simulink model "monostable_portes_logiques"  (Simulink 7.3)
settings: Solver=ode15s  StartTime=0.0  StopTime=1  RelTol=1e-3
StopFcn:
  | close all, clc
  | load signaux.mat
  | plot(x(1,:),x(2,:))
  | grid
  | title('Oscillateur à portes NAND, T=2RC ln3')
  | 
  | xlabel('temps')
  | axis([0 1 -0.1 1.1])
undefined symbols (not defined in the file or in its folder): sigbuilder_block
libraries: fl_lib x6, elec_lib x5, nesl_utility x4

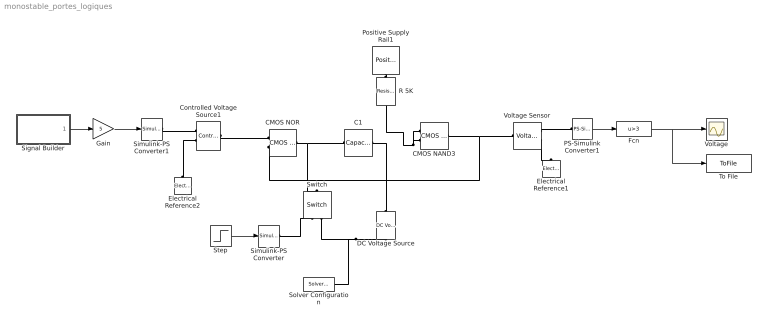
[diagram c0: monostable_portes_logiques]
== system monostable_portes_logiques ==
  C1 : fl_lib/Electrical/Electrical Elements/Capacitor  DialogController=NetworkEngine.DynNeDlgSource  SystemSampleTime=-1  c=100e-9 F  v0=0 V  r=1e-6 Ohm  g=0 1/Ohm  i_Log=off  v_Log=off  vc_Log=off  LocalVarNames=|current|voltage|power  LocalVarDescs=|Capacitor current (A)|Voltage across capacitor (V)|Power (W)  LocalVarLogging=[0 0 0]
  CMOS NAND3 : elec_lib/Integrated Circuits/Logic/CMOS NAND  DialogController=NetworkEngine.DynNeDlgSource  SystemSampleTime=-1  V_IL=2 V  V_IH=3 V  V_OL=0 V  V_OH=5 V  C_IN=5 pF  R_OUT=450 Ohm  Delay=1.2e-07 s  LocalVarLogging=[]
  CMOS NOR : elec_lib/Integrated Circuits/Logic/CMOS NOR  DialogController=NetworkEngine.DynNeDlgSource  SystemSampleTime=-1  V_IL=2 V  V_IH=3 V  V_OL=0 V  V_OH=5 V  C_IN=5 pF  R_OUT=450 Ohm  Delay=1.2e-07 s  LocalVarLogging=[]
  Controlled Voltage Source1 : fl_lib/Electrical/Electrical Sources/Controlled Voltage Source  DialogController=NetworkEngine.DynNeDlgSource  SystemSampleTime=-1  i_Log=off  v_Log=off  LocalVarNames=|current|voltage|power  LocalVarDescs=|Current (A)|Voltage (V)|Power (W)  LocalVarLogging=[0 0 0]
  DC Voltage Source : elec_lib/Sources/SPICE-Compatible Sources/DC Voltage Source  DialogController=NetworkEngine.DynNeDlgSource  SystemSampleTime=-1  DC=1 V  current_Log=off  voltage_Log=off  power_Log=off  LocalVarNames=|current|voltage|power  LocalVarDescs=|Current (A)|Voltage (V)|Power (W)  LocalVarLogging=[0 0 0]
  Electrical Reference1 : fl_lib/Electrical/Electrical Elements/Electrical Reference  DialogController=NetworkEngine.DynNeDlgSource  SystemSampleTime=-1  i_Log=off  LocalVarNames=|i  LocalVarDescs=|i  LocalVarLogging=[]
  Electrical Reference2 : fl_lib/Electrical/Electrical Elements/Electrical Reference  DialogController=NetworkEngine.DynNeDlgSource  SystemSampleTime=-1  i_Log=off  LocalVarNames=|i  LocalVarDescs=|i  LocalVarLogging=[]
  Fcn : Fcn  Expr=u>3
  Gain : Gain  Gain=5  ParameterDataType=fixdt(1, 16)  ParameterScaling=2^0  OutDataType=fixdt(1, 16)  OutScaling=2^0
  PS-Simulink Converter1 : nesl_utility/PS-Simulink Converter  DialogController=NetworkEngine.DynNeUtilDlgSource  SystemSampleTime=-1  PhysicalDomain=network_engine_domain  LeftPortType=input  RightPortType=output  SubClassName=ps_output  Unit=1  AffineConversion=off
  Positive Supply Rail1 : elec_lib/Sources/Positive Supply Rail  DialogController=NetworkEngine.DynNeDlgSource  SystemSampleTime=-1  v0=5 V  current_Log=off  voltage_Log=off  power_Log=off  LocalVarNames=|current|voltage|power  LocalVarDescs=|Current (A)|Voltage (V)|Power (W)  LocalVarLogging=[0 0 0]
  R 5K : elec_lib/Passive Devices/Resistor  DialogController=NetworkEngine.DynNeDlgSource  SystemSampleTime=-1  SCALE=1  R_param=1  R=5 kOhm  RSH=0 Ohm  LENGTH=1e-06 m  WIDTH=1e-06 m  NARROW=0 m  T_param=1  TC1=0 1/K  TC2=0 1/K^2  TOFFSET=0 K  TFIXED=300.15 K  TMEAS=300.15 K  LocalVarLogging=[]
  Signal Builder : Subsystem  Tag=STV Subsys  LoadFcn=sigbuilder_block('load',[198 37.5 550.5 399.75 ]);  StartFcn=sigbuilder_block('start');  StopFcn=sigbuilder_block('stop');  ClipboardFcn=sigbuilder_block('clipboard');
  Simulink-PS Converter : nesl_utility/Simulink-PS Converter  DialogController=NetworkEngine.DynNeUtilDlgSource  SystemSampleTime=-1  PhysicalDomain=network_engine_domain  LeftPortType=input  RightPortType=output  SubClassName=ps_input  Unit=1  AffineConversion=off  InputFilterTimeConstant=.001  UdotUserProvided=0
  Simulink-PS Converter1 : nesl_utility/Simulink-PS Converter  DialogController=NetworkEngine.DynNeUtilDlgSource  SystemSampleTime=-1  PhysicalDomain=network_engine_domain  LeftPortType=input  RightPortType=output  SubClassName=ps_input  Unit=1  AffineConversion=off  InputFilterTimeConstant=.001  UdotUserProvided=0
  Solver Configuration : nesl_utility/Solver Configuration  DialogController=NetworkEngine.DynNeUtilDlgSource  SystemSampleTime=-1  PhysicalDomain=network_engine_domain  LeftPortType=input  RightPortType=generic  SubClassName=solver  Accelerate=off  Profile=off  ResidualTolerance=1e-9  MaxNonlinIter=12  MaxModeIter=2  DoFixedCost=off  DoDC=off  LinearAlgebra=Sparse
  Step : Step  Time=0.001  Before=1  After=0  SampleTime=0
  Switch : fl_lib/Electrical/Electrical Elements/Switch  DialogController=NetworkEngine.DynNeDlgSource  SystemSampleTime=-1  R_closed=0.01 Ohm  G_open=1e-08 1/Ohm  i_Log=off  v_Log=off  LocalVarNames=|i|v  LocalVarDescs=|i|v  LocalVarLogging=[0 0]
  To File : ToFile  Filename=signaux  MatrixName=x
  Voltage : Scope
  Voltage Sensor : fl_lib/Electrical/Electrical Sensors/Voltage Sensor  DialogController=NetworkEngine.DynNeDlgSource  SystemSampleTime=-1  i1_Log=off  v1_Log=off  LocalVarNames=|i1|v1  LocalVarDescs=|i1|v1  LocalVarLogging=[0 0]
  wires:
  Step/1 -> Simulink-PS Converter/1
  PS-Simulink Converter1/1 -> Fcn/1
  Fcn/1 -> Voltage/1, To File/1
  Signal Builder/1(Signal 2) -> Gain/1
  Gain/1 -> Simulink-PS Converter1/1
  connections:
  Voltage Sensor/LConn1 -- CMOS NAND3/RConn1 -- CMOS NOR/LConn2
  Voltage Sensor/RConn2 -- Electrical Reference1/LConn1
  Voltage Sensor/RConn1 -- PS-Simulink Converter1/LConn1
  Switch/RConn2 -- DC Voltage Source/RConn1 -- Solver Configuration/RConn1
  Simulink-PS Converter/RConn1 -- Switch/RConn1
  DC Voltage Source/LConn1 -- C1/LConn1
  CMOS NOR/RConn1 -- C1/RConn1 -- Switch/LConn1
  CMOS NAND3/LConn1 -- CMOS NAND3/LConn2 -- R 5K/RConn1
  Positive Supply Rail1/RConn1 -- R 5K/LConn1
  Electrical Reference2/LConn1 -- Controlled Voltage Source1/RConn2
  Controlled Voltage Source1/LConn1 -- CMOS NOR/LConn1
  Simulink-PS Converter1/RConn1 -- Controlled Voltage Source1/RConn1

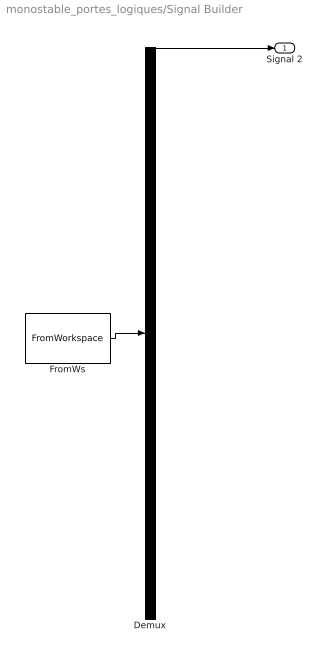
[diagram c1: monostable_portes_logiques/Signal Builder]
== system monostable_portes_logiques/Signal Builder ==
  Demux : Demux  Tag=STV Demux  Outputs=1
  FromWs : FromWorkspace  Tag=STV FromWs  VariableName=tuvar  SampleTime=0  SigBuilderData=DataTag0  VnvData=DataTag1
  Signal 2 : Outport  Tag=STV Outport
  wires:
  Demux/1 -> Signal 2/1
  FromWs/1 -> Demux/1
